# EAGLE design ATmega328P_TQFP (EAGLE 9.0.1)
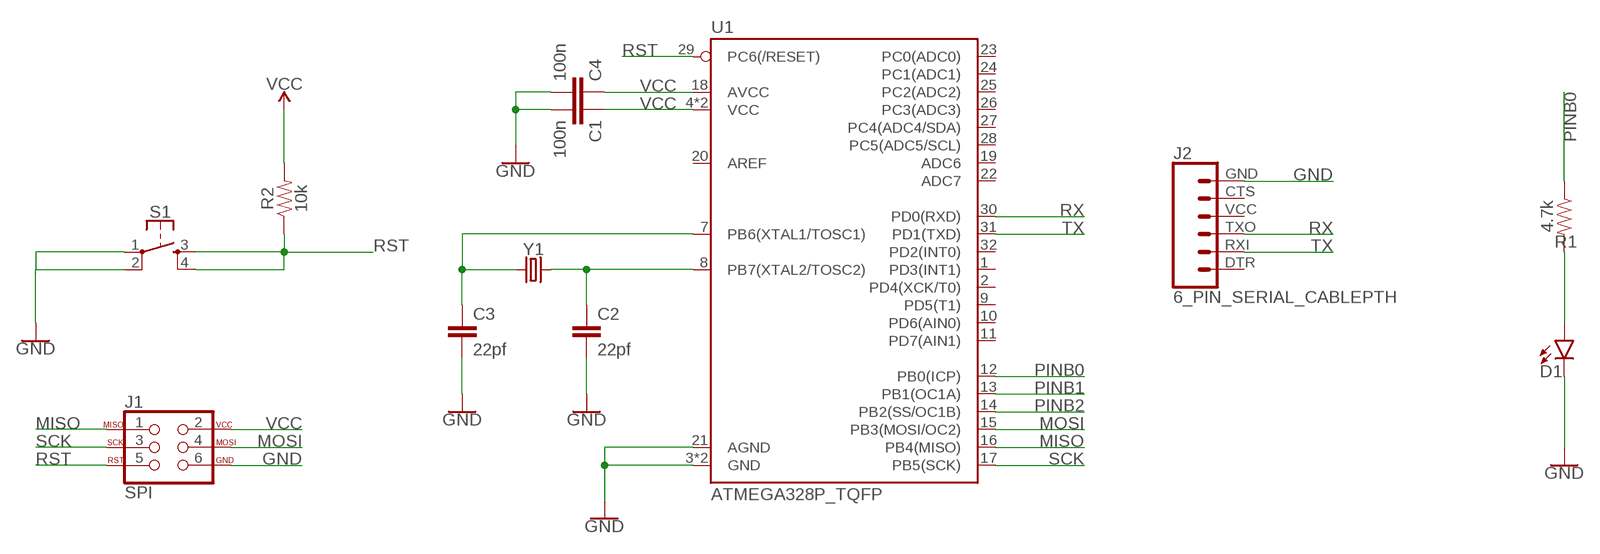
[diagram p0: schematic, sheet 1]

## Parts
C1  100n  2.2UF-0805-25V-(+80/-20%)  [0805]
C2  22pf  2.2UF-0805-25V-(+80/-20%)  [0805]
C3  22pf  2.2UF-0805-25V-(+80/-20%)  [0805]
C4  100n  2.2UF-0805-25V-(+80/-20%)  [0805]
D1  LED-FKIT-1206  [FKIT-LED-1206]
J1  SPI  AVR_SPI_PROG_3X2PTH  [2X3]
J2  6_PIN_SERIAL_CABLEPTH  [FTDI_BASIC]
R1  4.7k  0.22OHM-0805-1/4W-1%  [0805]
R2  10k  0.22OHM-0805-1/4W-1%  [0805]
S1  MOMENTARY-SWITCH-SPST-2-SMD-5.2MM  [TACTILE_SWITCH_SMD_5.2MM]
U1  ATMEGA328P_TQFP  [TQFP32-08]
Y1  CRYSTALSMD-5X3.2-4PAD  [CRYSTAL-SMD-5X3.2-4PAD]

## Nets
GND: C1.2 C2.2 C3.2 C4.2 D1.C J1.6 J2.GND S1.1 S1.2 U1.3(GND) U1.5(GND) U1.21(AGND)
MISO: J1.1 U1.16(PB4(MISO))
MOSI: J1.4 U1.15(PB3(MOSI/OC2))
N$1: C2.1 U1.8(PB7(XTAL2/TOSC2)) Y1.3
N$2: C3.1 U1.7(PB6(XTAL1/TOSC1)) Y1.1
N$4: D1.A R1.2
PINB0: R1.1 U1.12(PB0(ICP))
PINB1: U1.13(PB1(OC1A))
PINB2: U1.14(PB2(SS/OC1B))
RST: J1.5 R2.1 S1.3 S1.4 U1.29(PC6(/RESET))
RX: J2.TXO U1.30(PD0(RXD))
SCK: J1.3 U1.17(PB5(SCK))
TX: J2.RXI U1.31(PD1(TXD))
VCC: C1.1 C4.1 J1.2 R2.2 U1.4(VCC) U1.6(VCC) U1.18(AVCC)
Unconnected: J2.CTS J2.DTR J2.VCC U1.1(PD3(INT1)) U1.2(PD4(XCK/T0)) U1.9(PD5(T1)) U1.10(PD6(AIN0)) U1.11(PD7(AIN1)) U1.19(ADC6) U1.20(AREF) U1.22(ADC7) U1.23(PC0(ADC0)) U1.24(PC1(ADC1)) U1.25(PC2(ADC2)) U1.26(PC3(ADC3)) U1.27(PC4(ADC4/SDA)) U1.28(PC5(ADC5/SCL)) U1.32(PD2(INT0))

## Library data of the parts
C1-C4 = SparkFun-Capacitors:2.2UF: 2.2µF ceramic capacitors; PROD_ID: CAP-11624; VALUE: 2.2uF
D1 = SparkFun-LED:LED: LED (Generic)
J1 = SparkFun-Connectors:AVR_SPI_PROG_3X2: AVR ISP 6 Pin This is the reduced ISP connector for AVR programming. Common on Arduino. This footprint will take up less PCB space and can be used with a 10-pin to 6-pin adapter such as SKU: BOB-08508 **Special note about "TEST_POINT" package. The stop mask is on the top side, so if you want your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
J2 = SparkFun-Connectors:6_PIN_SERIAL_CABLE: 6-pin header connection for use with the "FTDI BASIC" pinout - CABLE SIDE. Also known as "Arduino Serial Program Header". This is used on a design to provide a 6-pin connection point for serial communication usually from a USB cable (D+/D-) to these headers (RX/TX). It also has the remaining pins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
R1 R2 = SparkFun-Resistors:0.22OHM: 0.22Ω resistor; PROD_ID: RES-09883; VALUE: 0.22
S1 = SparkFun-Switches:MOMENTARY-SWITCH-SPST-2: Momentary Switch (Pushbutton) - SPST - Two Circuits Normally-open (NO) SPST momentary switches (buttons, pushbuttons). Schematic symbol includes two switch circuits. Variants SMD-4.6MMX2.8MM - 4.60mm x 2.80mm Tactile Momentary Button Switch - Used on SparkFun SAMD21 Mini Breakout SMD-5.2MM - Mini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; PROD_ID: SWCH-08247; SF_SKU: COM-08720
U1 = SparkFun-IC-Microcontroller:ATMEGA328P_TQFP: Popular 328P in QFP Storefront component: ATmega328 - TQFP (COM-13448) Datasheet SparkFun Products SparkFun RedBoard - Programmed with Arduino (DEV-12757) Arduino Pro Mini 328 - 5V/16MHz (DEV-11113) Arduino Pro Mini 328 - 3.3V/8MHz (DEV-11114) SparkFun OpenLog (DEV-13712) SparkFun MicroView - OLED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; PROD_ID: IC-09069
Y1 = SparkFun-Clocks:CRYSTAL: Crystals (Generic)

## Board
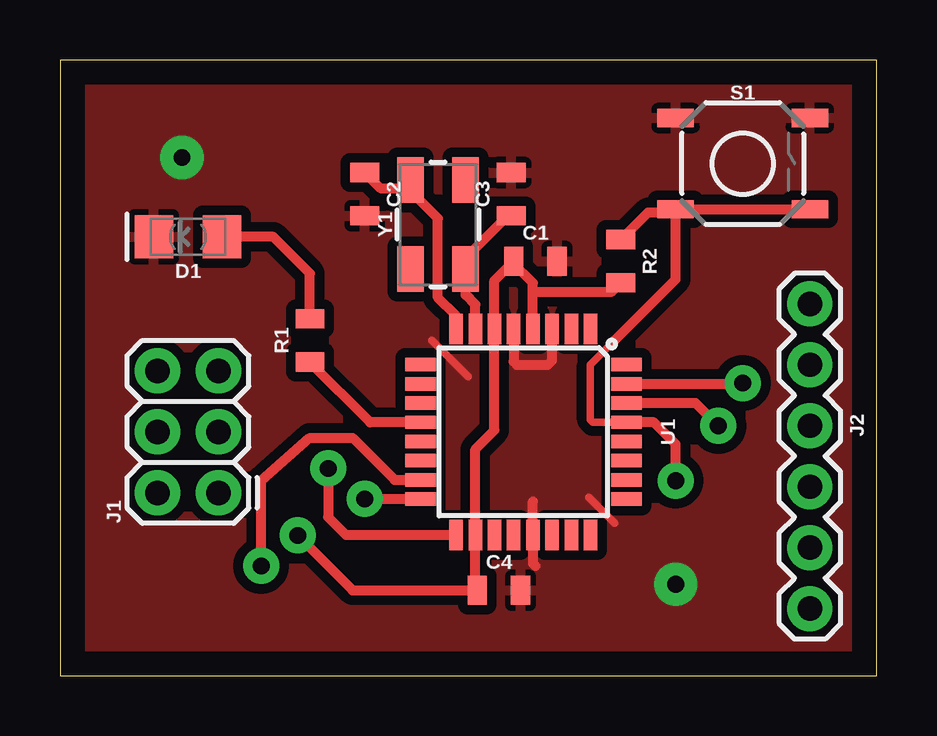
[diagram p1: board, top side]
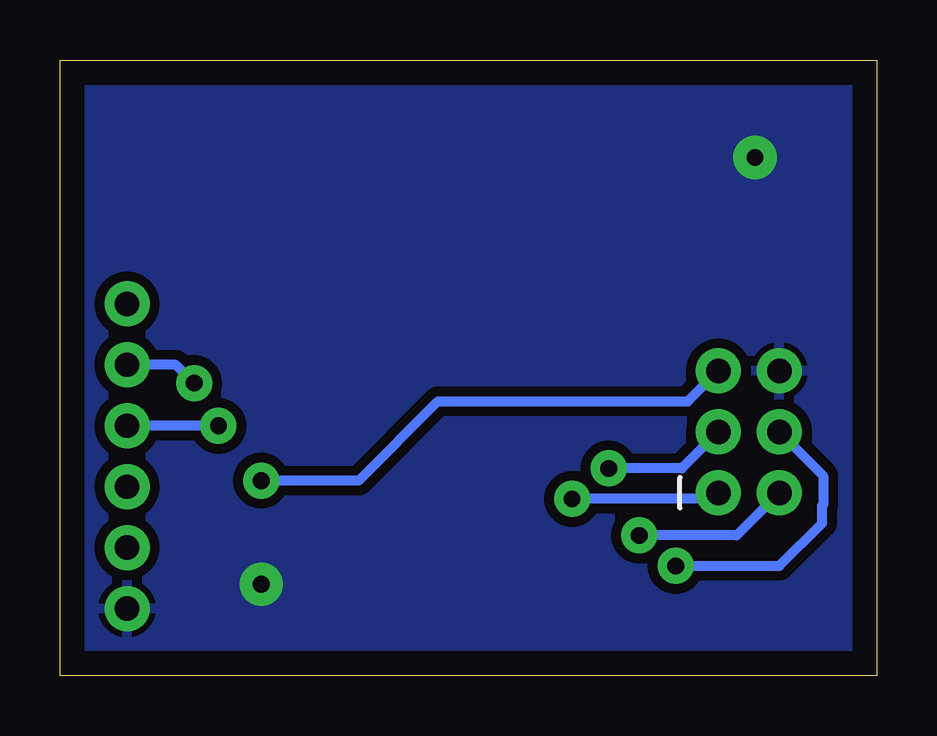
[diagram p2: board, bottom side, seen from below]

Size 34.04 x 25.65 mm. Coordinates in mm from the lower left corner, seen from the top.
Outline: 0,0 34.04,0 34.04,25.65 0,25.65 0,0
Copper layers (1*16): Top 0.035mm / dielectric 1.5mm / Bottom 0.035mm
Design rules "default": minimum track width 6mil, minimum drill 0.35mm, track to track 6mil, track to pad 6mil, pad to pad 6mil, via to via 6mil, smd to smd 6mil, copper to edge 40mil, drill to drill 6mil, minimum pad ring 10mil, minimum via ring 8mil, stop-mask expansion 4mil, vias tented up to drill 0mil, thermal gap 10mil
tRestrict: area 3.3,12 to 4.8,13.4; area 30.5,2.1 to 32,3.5

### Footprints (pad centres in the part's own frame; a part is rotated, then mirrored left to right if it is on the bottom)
0805 = smd 0.8 x 1.2: 1 -0.9,0; 2 0.9,0
FKIT-LED-1206 = smd 1.6 x 1.803: A -1.422,0; C 1.422,0
2X3 = drill 1.016 pad 1.88: 1 0,0; 2 0,2.54; 3 2.54,0; 4 2.54,2.54; 5 5.08,0; 6 5.08,2.54
FTDI_BASIC = drill 1.016 pad 1.88: CTS 10.16,0; DTR 0,0; GND 12.7,0; RXI 2.54,0; TXO 5.08,0; VCC 7.62,0
TACTILE_SWITCH_SMD_5.2MM = smd 1.524 x 0.762: 1 -2.794,1.905; 2 2.794,1.905; 3 -2.794,-1.905; 4 2.794,-1.905
TQFP32-08 = smd 1.27 x 0.559: 1 -4.293,2.8; 2 -4.293,2; 3 -4.293,1.2; 4 -4.293,0.4; 5 -4.293,-0.4; 6 -4.293,-1.2; 7 -4.293,-2; 8 -4.293,-2.8; 17 4.293,-2.8; 18 4.293,-2; 19 4.293,-1.2; 20 4.293,-0.4; 21 4.293,0.4; 22 4.293,1.2; 23 4.293,2; 24 4.293,2.8 | smd 0.559 x 1.27: 9 -2.8,-4.293; 10 -2,-4.293; 11 -1.2,-4.293; 12 -0.4,-4.293; 13 0.4,-4.293; 14 1.2,-4.293; 15 2,-4.293; 16 2.8,-4.293; 25 2.8,4.293; 26 2,4.293; 27 1.2,4.293; 28 0.4,4.293; 29 -0.4,4.293; 30 -1.2,4.293; 31 -2,4.293; 32 -2.8,4.293
CRYSTAL-SMD-5X3.2-4PAD = smd 1.9 x 1.1: 1 -1.85,-1.15; 2 1.85,-1.15; 3 1.85,1.15; 4 -1.85,1.15

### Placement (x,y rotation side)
C1  19.81,17.27 0 top
C2  12.7,20.07 270 top
C3  18.8,20.07 90 top
C4  18.29,3.56 0 top
D1  5.33,18.29 180 top
J1  6.6,7.62 90 top
J2  31.24,15.49 270 top
R1  10.41,13.97 90 top
R2  23.37,17.27 270 top
S1  28.45,21.34 0 top
U1  19.3,10.16 270 top
Y1  15.75,18.8 90 top

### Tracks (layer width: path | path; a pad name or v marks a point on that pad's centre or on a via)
GND  (via drill 0.7 pad 1.8)
  Top 0.305: 22.03,7.44 23.11,6.35 | 17.02,12.45 15.49,13.97
  Top 0.406: 19.81,4.57 19.7,4.68 U1.21 19.7,7.26 | 20.57,14.52 U1.3 20.5,13.14 20.32,12.95 19.05,12.95 18.9,13.1 U1.5
  other vias: 5.08,21.59 25.65,3.81
  pour Top (isolate 0.406): 0,0 34.04,0 34.04,25.65 0,25.65
  pour Bottom (isolate 0.406): 0,0 34.04,0 34.04,25.65 0,25.65
MISO  (via drill 0.7 pad 1.5)
  Top 0.406: v12.7,7.37 U1.16
  Bottom 0.406: J1.1 6.86,7.37 v12.7,7.37
MOSI  (via drill 0.7 pad 1.5)
  Top 0.406: U1.15 13.94,8.16 12.19,9.91 10.41,9.91 8.38,8.13 v8.38,4.57
  Bottom 0.406: J1.4 2.23,8.33 2.23,7.11 2.29,7.06 2.29,6.35 4.06,4.57 v8.38,4.57
N$1
  Top 0.254: 14.85,20.2 14.85,20.32 14.85,20.45 Y1.3
  Top 0.406: U1.8 16.5,14.99 15.75,15.75 15.75,19.05 14.85,19.95 14.85,20.2 | C2.1 13.35,20.32 14.85,20.32
N$2
  Top 0.406: 17.15,16.38 Y1.1 | Y1.1 17.15,17.52 | U1.7 17.3,15.46 16.9,15.87 Y1.1 | Y1.1 16.9,17.41 18.66,19.17 C3.1
N$4
  Top 0.406: R1.2 10.41,16.76 8.89,18.29 D1.A
PINB0
  Top 0.406: U1.12 12.92,10.56 R1.1
RST  (via drill 0.7 pad 1.5)
  Top 0.305: U1.29 22.21,10.56 22.1,10.67 22.1,12.95 23.11,13.97
  Top 0.406: v25.65,8.13 25.65,9.65 24.75,10.56 U1.29 | 23.11,13.97 25.65,16.51 25.65,19.3 | 25.65,19.3 S1.3 S1.4 | R2.1 24.5,19.3 25.65,19.3
  Bottom 0.406: v25.65,8.13 21.59,8.13 18.29,11.43 7.87,11.43 J1.5
RX  (via drill 0.7 pad 1.5)
  Top 0.406: v27.43,10.41 26.49,11.36 U1.30
  Bottom 0.406: v27.43,10.41 J2.TXO
SCK  (via drill 0.7 pad 1.5)
  Top 0.406: v11.18,8.64 11.18,6.6 11.91,5.87 U1.17
  Bottom 0.406: J1.3 8.13,8.64 v11.18,8.64
TX  (via drill 0.7 pad 1.5)
  Top 0.406: v28.45,12.19 28.42,12.16 U1.31
  Bottom 0.406: J2.RXI 29.21,12.95 v28.45,12.19
VCC  (via drill 0.7 pad 1.5)
  Top 0.406: 17.27,3.56 C4.1 17.3,3.64 U1.18 17.3,9.43 18.1,10.23 U1.6 18.1,16.46 18.85,17.21 | v9.91,5.84 12.19,3.56 17.27,3.56 | 17.27,3.56 17.3,3.59 | 18.85,17.21 C1.1 | 18.85,17.21 19.7,16.36 19.7,16 | U1.4 19.7,16 | R2.2 23,16 19.7,16
  Bottom 0.406: J1.2 5.84,5.84 v9.91,5.84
